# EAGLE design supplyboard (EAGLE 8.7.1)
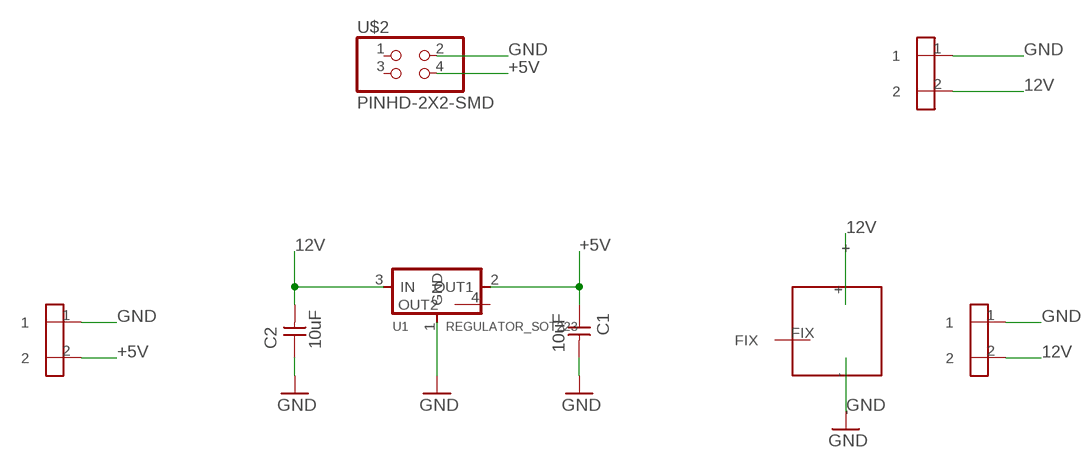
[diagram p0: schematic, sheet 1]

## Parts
C1  10uF  CAP-UNPOLARIZEDFAB  [C1206FAB]
C2  10uF  CAP-UNPOLARIZEDFAB  [C1206FAB]
DCJACK1  AKIZUKI_DCJACK  [AKIZUKI_DCJACK]
TML1  AKIZUKITNK_HOLE2PIN  [5.08PICH_HL]
TML2  AKIZUKITNK_HOLE2PIN  [5.08PICH_HL]
TML3  AKIZUKITNK_HOLE2PIN  [5.08PICH_HL]
U1  REGULATOR_SOT223  [SOT223]
U$2  PINHD-2X2-SMD  [2X02SMD]

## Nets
12V: C2.2 DCJACK1.+ TML1.2 TML3.2 U1.3(IN)
+5V: C1.1 TML2.2 U1.2(OUT1) U$2.4
GND: C1.2 C2.1 DCJACK1.- TML1.1 TML2.1 TML3.1 U1.1(GND) U$2.2
Unconnected: DCJACK1.FIX U1.4(OUT2) U$2.1 U$2.3

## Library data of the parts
C1 C2 = fab:CAP-UNPOLARIZED
DCJACK1 = doyo:AKIZUKI_DCJACK
TML1-TML3 = doyo:AKIZUKI?TNK_HOLE2PIN
U1 = fab:REGULATOR_SOT223
U$2 = fab:PINHD-2X2-SMD

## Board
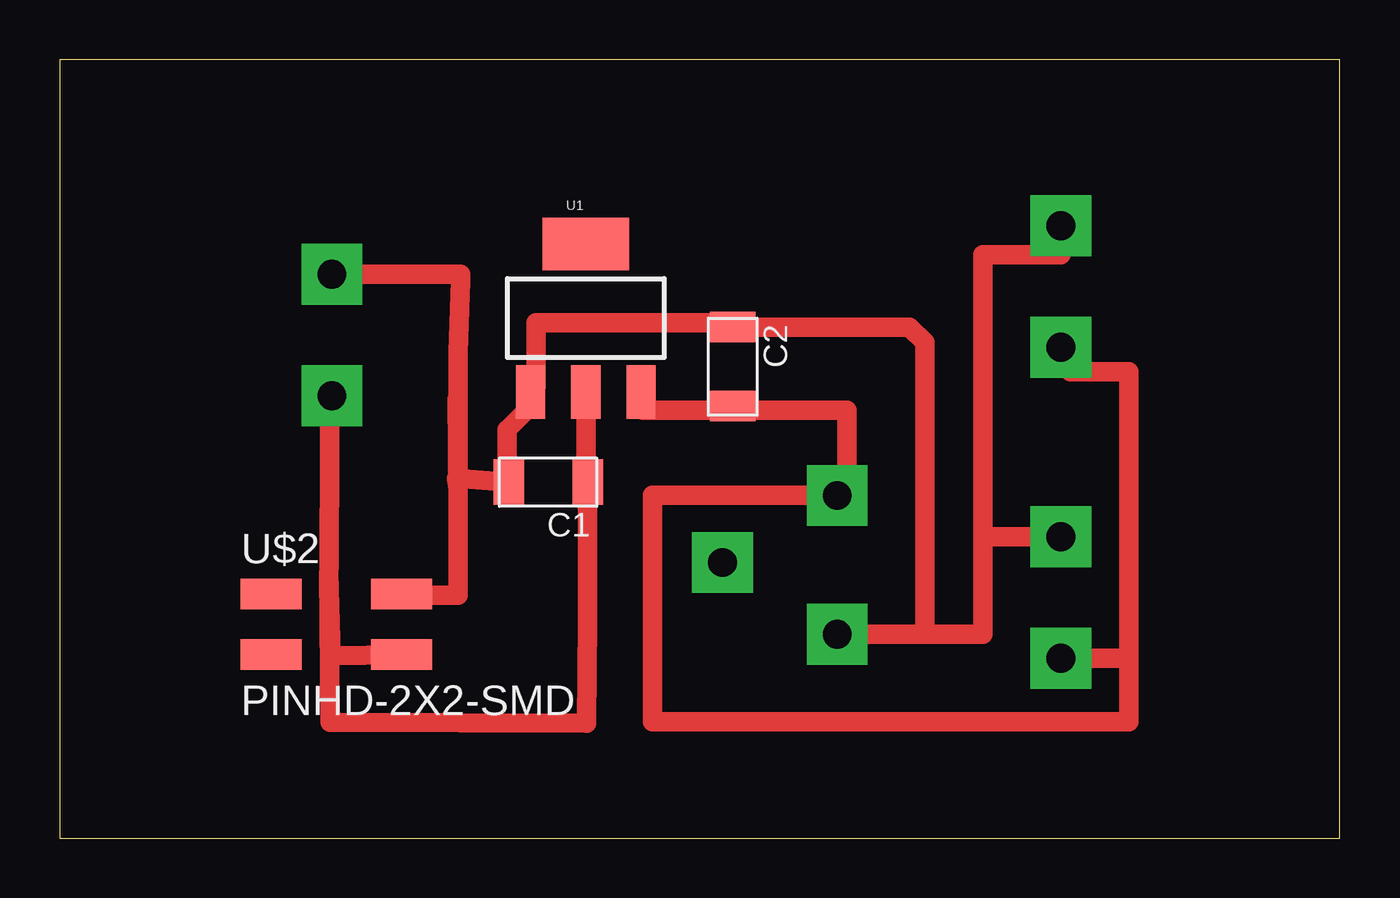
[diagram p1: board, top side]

Size 53.52 x 32.54 mm. Coordinates in mm from the lower left corner, seen from the top.
Outline: 0,0 53.52,0 53.52,32.54 0,32.54 0,0
Copper layers (1*16): Top 0.035mm / dielectric 1.5mm / Bottom 0.035mm
Design rules "default *": minimum track width 6mil, minimum drill 0.35mm, track to track 0.4mm, track to pad 0.4mm, pad to pad 0.4mm, via to via 0.4mm, smd to smd 0.4mm, copper to edge 40mil, drill to drill 6mil, minimum pad ring 10mil, minimum via ring 8mil, stop-mask expansion 4mil, vias tented up to drill 0mil, thermal gap 10mil

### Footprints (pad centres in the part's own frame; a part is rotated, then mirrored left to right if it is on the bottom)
C1206FAB = smd 1.27 x 1.905: 1 -1.651,0; 2 1.651,0
AKIZUKI_DCJACK = drill 1.2 pad 2.54 square: + 0,0; - 0,5.8; FIX 4.8,2.8
5.08PICH_HL = drill 1.2 pad 2.54 square: 1 0,0; 2 -5.08,0
SOT223 = smd 1.219 x 2.235: 1 -2.311,-3.099; 2 0,-3.099; 3 2.311,-3.099 | smd 3.6 x 2.2: 4 0,3.099
2X02SMD = smd 2.54 x 1.27: 1 -2.54,1.27; 2 2.92,1.27; 3 -2.54,-1.27; 4 2.92,-1.27

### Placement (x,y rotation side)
C1  20.42,14.88 180 top
C2  28.14,19.71 270 top
DCJACK1  32.51,14.33 180 top
TML1  41.86,25.6 90 top
TML2  11.38,23.57 90 top
TML3  41.86,12.6 90 top
U1  22,21.74 0 top
U$2  11.38,8.94 0 top

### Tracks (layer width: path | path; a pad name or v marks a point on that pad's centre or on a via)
12V
  Top 0.813: C2.2 28.35,17.86 | C2.2 27.96,17.88 24.38,17.88 24.38,18.57 U1.3 | C2.2 28.32,17.88 32.92,17.88 32.92,14.73 DCJACK1.+ 24.79,14.33 24.79,4.88 44.7,4.88 44.7,7.52 | 44.7,7.52 44.7,19.51 42.27,19.51 TML1.2 | TML3.2 44.7,7.52
+5V
  Top 0.813: U1.2 22,14.4 C1.1 22.07,9.07 22.02,4.8 11.3,4.85 11.25,11.07 | 11.25,11.07 11.35,7.62 U$2.4 | 11.25,11.07 11.25,10.62 11.27,11.78 11.28,15.85 11.28,18.49 TML2.2
GND
  Top 0.813: 16.66,14.63 16.59,15.04 C1.2 18.69,14.96 18.69,17.07 19.68,18.06 U1.1 19.91,18.87 19.91,21.54 27.96,21.54 C2.1 35.53,21.36 36.17,20.73 36.17,8.53 | 16.66,14.22 16.61,18.34 | 16.66,14.63 16.66,14.22 | 16.66,14.22 16.66,10.16 14.35,10.16 U$2.2 | 16.66,14.63 16.66,20.32 16.76,23.29 16.76,23.57 TML2.1 | DCJACK1.- 32.52,8.53 36.17,8.53 | 36.17,8.53 38.61,8.53 38.61,12.6 | 38.61,12.6 38.61,24.38 41.86,24.38 TML1.1 | TML3.1 38.61,12.6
